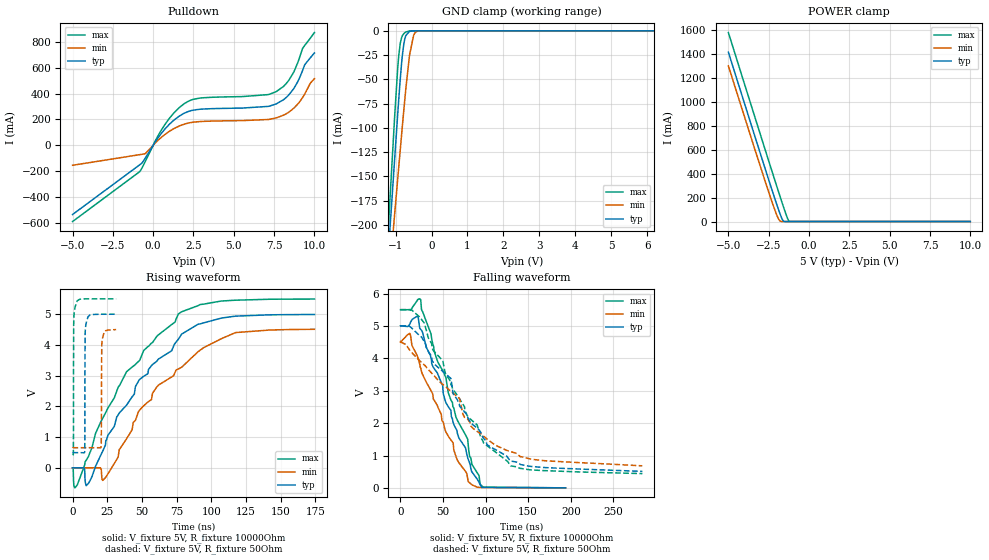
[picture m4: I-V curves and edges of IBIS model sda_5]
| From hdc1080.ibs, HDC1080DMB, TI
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|   sda_5 Model
[Model]   sda_5
Model_type   I/O_open_drain
Polarity   Non-Inverting
Vinl = 1.5
Vinh = 3.5
Vmeas = 2.5
Vref = 5
Cref = 2pF
Rref = 10000
|   typ   min   max
|   (nom PVT)   (fast PVT)   (slow PVT)
C_comp   3.555e-12   3.494e-12   3.618e-12
[Model spec]
|subparameter
Vinl   1.5   1.35   1.65
Vinh   3.5   3.15   3.85
| Where nom  PVT is Nominal Process, 5V, 27C
|   Fast PVT is Strong Process,  5.5V, -40C
|   Slow PVT is Weak Process,   4.5V, 150C
[Voltage Range]   5   4.5   5.5
|Junction Temperature
[Temperature Range]   27   150   -40
[Pullup Reference]   5   4.5   5.5
[Pulldown Reference]   0   0   0
[Power Clamp Reference]   5   4.5   5.5
[GND Clamp Reference]   0   0   0
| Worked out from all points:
|   slope of the pulldown table from 0 to 0.75 V, typ, clamps not added: 5.82 ohm
|   GND clamp passes 1 mA (typ) near -0.62 V on its own axis
|   POWER clamp passes 1 mA (typ) near -1.54 V on its own axis
|   falling waveform, V_fixture 5V, R_fixture 10000Ohm: 20-80 % time 42.3ns typ, 41.5ns min, 42ns max; typ from 5 V to 0.002 V
|   rising waveform, V_fixture 5V, R_fixture 10000Ohm: 20-80 % time 48ns typ, 48.1ns min, 47.3ns max; typ from 0.002 V to 4.99 V
|   falling waveform, V_fixture 5V, R_fixture 50Ohm: 20-80 % time 65.4ns typ, 74.7ns min, 60.8ns max; typ from 5 V to 0.51 V
|   rising waveform, V_fixture 5V, R_fixture 50Ohm: 20-80 % time 163ps typ, 218ps min, 145ps max; typ from 0.497 V to 5 V
[Pulldown]
|   Voltage   I(typ)   I(min)   I(max)
-5V       -535.1mA   -154.2mA   -589.6mA
-830mV    -150mA     -71.91mA   -203mA
-500mV    -100.5mA   -65.4mA    -127.1mA
700mV     121.9mA    81.44mA    155.9mA
1.849V    243.3mA    160.5mA    315.1mA
2.87V     278.8mA    183.7mA    365.1mA
7.639V    321mA      212.6mA    416.3mA
8.261V    371.5mA    244.9mA    479.4mA
8.734V    442.1mA    288.9mA    571.3mA
9.261V    577.7mA    368.6mA    748.8mA
9.41V     625.6mA    399.5mA    775mA
10V       714.3mA    516.3mA    872.2mA
[GND Clamp]
|   Voltage   I(typ)   I(min)   I(max)
-5V       -1.812A    -1.666A    -1.926A
-1.53V    -409.8mA   -411.6mA   -416.6mA
-1.024V   -131.2mA   -188.1mA   -87.37mA
-940mV    -85.77mA   -152.6mA   -38.5mA
-869.5mV  -49.88mA   -122.8mA   -12.88mA
-825.5mV  -30.71mA   -104.4mA   -6.288mA
-775mV    -14.7mA    -83.68mA   -3.106mA
-715mV    -4.847mA   -59.96mA   -1.22mA
-612.5mV  -597.8uA   -25.38mA   -109uA
-500mV    -41.16uA   -4.972mA   -3.075uA
-369.5mV  -1.045uA   -251.7uA   -21.31nA
10V       0A         0A         0A
[POWER Clamp]
|   Voltage   I(typ)   I(min)   I(max)
-5V       1.417A     1.303A     1.582A
-2.732V   447.7mA    342.6mA    606.8mA
-2.043V   160.8mA    69.82mA    314mA
-1.922V   112.2mA    30.38mA    262.8mA
-1.823V   73.97mA    8.2mA      221.4mA
-1.695V   29mA       400.4uA    168.3mA
-1.61V    7.428mA    37.84uA    133.4mA
-1.36V    914.4nA    0A         36.34mA
-1.238V   0A         0A         3.593mA
10V       0A         0A         0A
[Ramp]
R_load = 10000
|   typ   min   max
dV/dt_r   2.99821/4.80278e-08   2.71077/4.79577e-08   3.29849/4.7094e-08
dV/dt_f   2.99843/4.2251e-08   2.71108/4.1617e-08   3.29863/4.19235e-08
[Falling Waveform]
V_fixture = 5V
V_fixture_min = 4.5V
V_fixture_max = 5.5V
R_fixture = 10000Ohm
|   Time   V(typ)   V(min)   V(max)
0s        5V         4.5V       5.5V
10.95ns   5.054V     4.768V     5.5V
20.24ns   5.298V     4.035V     5.81V
23.81ns   4.89V      3.698V     5.801V
39.44ns   3.689V     2.714V     4.235V
66.83ns   1.682V     855.9mV    2.087V
78.93ns   933.8mV    290.9mV    1.504V
81.2ns    768.8mV    158.3mV    974.6mV
93.55ns   105.3mV    15.47mV    110.7mV
193.8ns   2.481mV    3.345mV    2.139mV
[Rising Waveform]
V_fixture = 5V
V_fixture_min = 4.5V
V_fixture_max = 5.5V
R_fixture = 10000Ohm
|   Time   V(typ)   V(min)   V(max)
0s        2.463mV    3.321mV    2.127mV
1.977ns   2.463mV    3.321mV    -639.6mV
8.36ns    2.665mV    3.321mV    47.87mV
10.01ns   -573.4mV   3.321mV    261.9mV
20.16ns   398.6mV    3.511mV    1.481V
21.89ns   562.7mV    -401.5mV   1.629V
47.79ns   2.846V     1.846V     3.477V
76.2ns    4.183V     3.218V     5.009V
117.4ns   4.938V     4.403V     5.457V
174.3ns   4.991V     4.511V     5.494V
[Falling Waveform]
V_fixture = 5V
V_fixture_min = 4.5V
V_fixture_max = 5.5V
R_fixture = 50Ohm
|   Time   V(typ)   V(min)   V(max)
0s        5V         4.5V       5.5V
27.89ns   4.514V     3.799V     5.091V
38.37ns   3.88V      3.497V     4.246V
49.76ns   3.594V     3.193V     3.926V
59.16ns   3.38V      2.985V     3.193V
62.74ns   2.849V     2.906V     3.003V
75.04ns   2.352V     2.181V     2.513V
97.6ns    1.532V     1.596V     1.388V
129.3ns   831.3mV    1.122V     680.3mV
284.1ns   510.1mV    681.5mV    441.5mV
[Rising Waveform]
V_fixture = 5V
V_fixture_min = 4.5V
V_fixture_max = 5.5V
R_fixture = 50Ohm
|   Time   V(typ)   V(min)   V(max)
0s        496.7mV    657.5mV    431.7mV
596ps     496.7mV    657.5mV    500.8mV
858ps     496.7mV    657.5mV    4.75V
2.13ns    496.7mV    657.5mV    5.278V
8.722ns   511.7mV    657.5mV    5.499V
9.1ns     4.363V     657.5mV    5.5V
10.25ns   4.793V     657.5mV    5.5V
20.51ns   5V         670mV      5.5V
21.21ns   5V         4.118V     5.5V
31.38ns   5V         4.5V       5.5V
